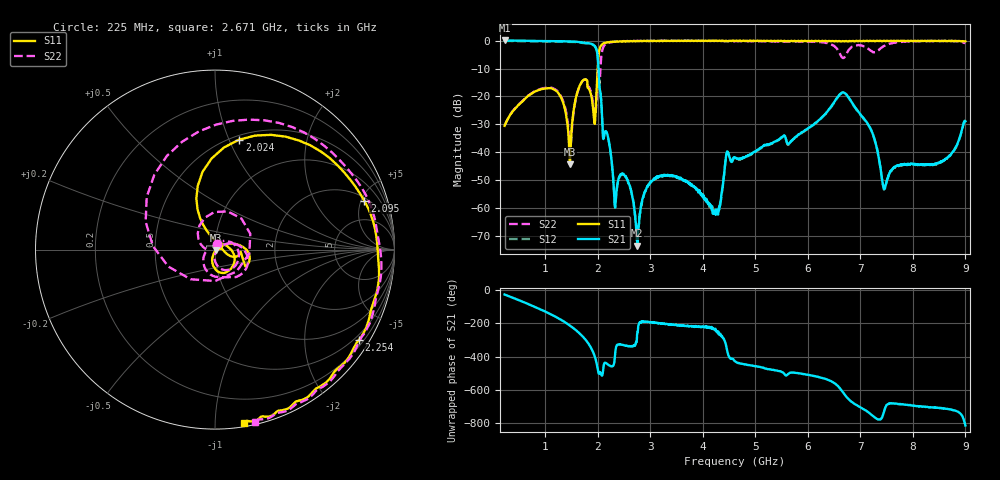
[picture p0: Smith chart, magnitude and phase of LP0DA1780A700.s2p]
!Agilent Technologies,E8358A,US41080443,A.07.50.56
!Agilent E8358A: A.07.50.56
!Date: Wednesday, August 24, 2016 14:55:17
!Correction: S11(Full 2 Port(1,2))
!S21(Full 2 Port(1,2))
!S12(Full 2 Port(1,2))
!S22(Full 2 Port(1,2))
!S2P File: Measurements: S11, S21, S12, S22:
# Hz S  dB  R 50
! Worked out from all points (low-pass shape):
!   1601 points, 225 MHz to 9 GHz, reference 50 ohm
!   highest |S21| = 0.04 dB at 225 MHz (marker M1); lowest = -73.4 dB at 2.753 GHz (marker M2)
!   |S21| within 3 dB of the highest: start of sweep to 1.971 GHz
!   lowest |S11| = -44.3 dB at 1.47 GHz (marker M3), VSWR 1.01, Z = 50.5 - j0.335 ohm
!   |S11| at or under -10 dB: start of sweep to 1.998 GHz
!   |S22| runs from -39.4 to 0.0 dB; largest |S21 - S12| = 0.019
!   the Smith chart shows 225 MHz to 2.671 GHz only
!   S11 on the Smith chart (normalised r, x): 225 MHz: 1.03, +0.05; 2.024 GHz: 0.54, +1.09; 2.095 GHz: 2.28, +5.32; 2.254 GHz: 0.36, -3.43; 2.671 GHz: 0.03, -1.18
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2.25e8  -30.49 53.8  0.04 -27.6  -0.12 -27.3  -30.39 72.3
8.611875e8  -17.76 -34.0  -0.15 -109.4  -0.30 -109.2  -17.63 -5.1
1.469953e9  -44.33 -33.1  -0.29 146.5  -0.44 146.7  -38.62 -49.4
1.689328e9  -14.93 -1.9  -0.66 88.4  -0.80 88.7  -15.00 -8.4
1.881281e9  -20.26 -22.6  -1.21 6.9  -1.35 7.2  -19.53 -125.7
2.023875e9  -4.05 77.6  -14.33 -142.1  -14.44 -141.9  -14.30 -6.5
2.095172e9  -1.15 18.1  -33.16 -136.6  -33.33 -136.4  -2.81 82.2
2.254219e9  -0.49 -32.2  -41.57 -97.6  -41.72 -97.0  -0.57 -12.6
2.671031e9  -0.19 -80.5  -56.99 24.4  -56.87 25.8  -0.14 -77.0
2.753297e9  -0.14 -86.6  -73.38 107.1  -73.56 90.9  -0.11 -84.2
3.153656e9  -0.12 -106.2  -48.94 162.5  -48.79 161.5  -0.09 -110.1
4.250531e9  -0.03 -133.7  -60.40 114.0  -61.13 110.1  -0.12 -165.9
4.6125e9  -0.15 -140.0  -41.81 -67.4  -42.03 -67.6  -0.20 172.5
6.076828e9  -0.10 -173.0  -30.40 -153.2  -30.65 -153.1  -0.47 56.8
6.449766e9  -0.19 178.4  -23.44 172.5  -23.60 172.1  -1.39 2.5
6.603328e9  -0.18 174.1  -19.30 133.7  -19.46 134.5  -4.49 -67.7
6.723984e9  -0.17 172.1  -19.06 84.3  -19.23 84.5  -5.08 161.5
6.899484e9  -0.24 168.9  -23.92 35.9  -23.99 35.9  -1.75 68.7
7.102406e9  -0.13 164.3  -28.79 -1.6  -28.94 -2.1  -2.31 0.3
7.250484e9  -0.09 161.4  -34.12 -37.9  -34.27 -37.4  -4.20 -87.4
7.541156e9  -0.21 156.6  -48.08 38.4  -48.36 40.6  -1.25 131.3
9e9  -0.27 136.3  -28.87 -91.8  -29.00 -92.0  -0.90 47.9
